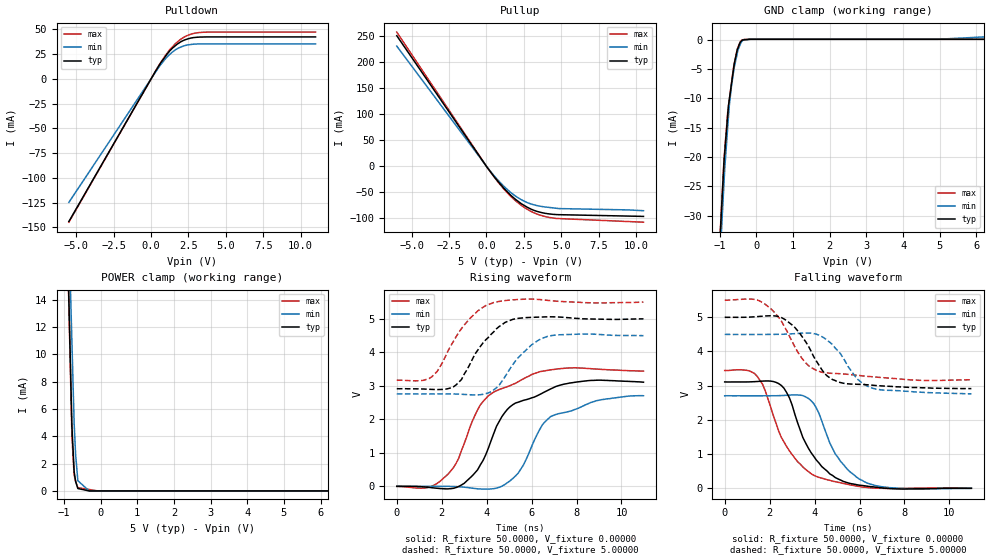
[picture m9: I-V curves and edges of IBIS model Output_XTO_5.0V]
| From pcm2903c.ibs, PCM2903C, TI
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[Model] Output_XTO_5.0V
Model_type Output
Vref  = 0.00000V
Cref  = 1.00000pF
Vmeas = 1.65000V
C_comp  2.00000pF 2.00000pF 2.00000pF
| variable   typ   min   max
[Voltage Range]   5.00000V  4.50000V  5.50000V
[POWER Clamp Reference]  5.00000V  4.50000V  5.50000V
[Pullup Reference]   5.00000V  4.50000V  5.50000V
[Pulldown Reference]   0.00000V  0.00000V  0.00000V
[GND Clamp Reference]   0.00000V  0.00000V  0.00000V
[Temperature Range]   25   85   -25
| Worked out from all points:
|   slope of the pulldown table from 0 to 0.75 V, typ, clamps not added: 40.8 ohm
|   slope of the pullup table from 0 to 0.75 V, typ, clamps not added: 26.9 ohm
|   GND clamp passes 1 mA (typ) near -0.48 V on its own axis
|   POWER clamp passes 1 mA (typ) near -0.70 V on its own axis
|   rising waveform, R_fixture 50.0000, V_fixture 0.00000: 20-80 % time 1.58ns typ, 1.62ns min, 1.54ns max; typ from 0 V to 3.11 V
|   falling waveform, R_fixture 50.0000, V_fixture 0.00000: 20-80 % time 1.37ns typ, 1.27ns min, 1.53ns max; typ from 3.11 V to 0 V
|   falling waveform, R_fixture 50.0000, V_fixture 5.00000: 20-80 % time 1.21ns typ, 1.2ns min, 1.3ns max; typ from 5 V to 2.92 V
|   rising waveform, R_fixture 50.0000, V_fixture 5.00000: 20-80 % time 1.28ns typ, 1.24ns min, 1.31ns max; typ from 2.92 V to 5 V
[GND Clamp]
-5V       -516.7mA   -511.3mA   -516.9mA
-881.1mV  -20.69mA   -24.2mA    -20.2mA
-861mV    -19.12mA   -21.83mA   -18.62mA
-780.2mV  -12.77mA   -14.83mA   -12.28mA
-760.1mV  -11.19mA   -13.08mA   -11.31mA
-739.6mV  -10.26mA   -11.31mA   -10.32mA
-679mV    -7.53mA    -7.887mA   -7.391mA
-623.5mV  -5.02mA    -5.556mA   -4.707mA
-522mV    -1.726mA   -2.33mA    -1.604mA
-380.7mV  -26.86uA   -130.3uA   -17.92uA
4.936V    100.6uA    99.12uA    98.92uA
10V       100.6uA    1.685mA    98.92uA
[Pulldown]
-5.5V     -144.1mA   -124.7mA   -144.7mA
279.4mV   7.251mA    6.327mA    7.216mA
658.9mV   16.41mA    14.59mA    16.72mA
1.063V    24.82mA    21.85mA    25.7mA
1.503V    31.88mA    27.93mA    33.47mA
1.902V    36.52mA    31.48mA    38.99mA
2.221V    39.05mA    33.32mA    42.17mA
2.6V      40.86mA    34.48mA    44.68mA
3.5V      42.18mA    35.22mA    46.98mA
11V       42.25mA    35.23mA    47.12mA
[Pullup]
-6V       250.4mA    230.5mA    257.3mA
39.2mV    -1.888mA   -1.438mA   -1.786mA
620.5mV   -23.75mA   -21.93mA   -24.46mA
1.121V    -40.74mA   -37.25mA   -42.2mA
1.621V    -55.47mA   -50.17mA   -57.51mA
2.081V    -66.41mA   -59.75mA   -69.29mA
2.698V    -78mA      -69.23mA   -81.85mA
3.139V    -83.99mA   -73.53mA   -88.61mA
3.557V    -87.78mA   -76.29mA   -93.35mA
4.301V    -91.58mA   -79.17mA   -98.42mA
4.837V    -92.68mA   -80.99mA   -100.1mA
10.5V     -95.98mA   -85.1mA    -107.1mA
[POWER Clamp]
-5V       474.9mA    423mA      493.3mA
-1.139V   44.73mA    45.92mA    45.58mA
-780.6mV  4.768mA    10.9mA     4.029mA
-719.7mV  1.418mA    4.948mA    1.152mA
-679.5mV  698.8uA    2.661mA    700.7uA
-618.7mV  176.3uA    747.4uA    239uA
-309.4mV  0A         0A         104.4uA
-38.05mV  0A         0A         0A
10V       0A         0A         0A
[Rising Waveform]
R_fixture = 50.0000
V_fixture = 0.00000
V_fixture_min = 0.00000
V_fixture_max = 0.00000
0s        0V         0V         0V
1.8ns     -57.41mV   546.8uV    89.3mV
2.52ns    -59.46mV   -4.152mV   557.5mV
3ns       89.55mV    -25.72mV   1.275V
3.72ns    642.5mV    -78.93mV   2.435V
4.44ns    1.795V     -52.7mV    2.856V
5.4ns     2.512V     389.9mV    3.123V
6.36ns    2.742V     1.698V     3.422V
6.84ns    2.907V     2.08V      3.478V
10.98ns   3.11V      2.705V     3.443V
[Falling Waveform]
R_fixture = 50.0000
V_fixture = 0.00000
V_fixture_min = 0.00000
V_fixture_max = 0.00000
0s        3.11V      2.705V     3.443V
1.44ns    3.122V     2.703V     3.279V
1.8ns     3.138V     2.706V     2.86V
2.52ns    3.007V     2.711V     1.489V
2.88ns    2.646V     2.724V     1.095V
3.96ns    937.5mV    2.48V      381.9mV
4.92ns    314.5mV    1.006V     192.3mV
6ns       89.87mV    266.5mV    50.41mV
7.32ns    -6.881mV   20.15mV    -4.144mV
10.98ns   0V         0V         0V
[Falling Waveform]
R_fixture = 50.0000
V_fixture = 5.00000
V_fixture_min = 4.50000
V_fixture_max = 5.50000
0s        5V         4.5V       5.5V
1.56ns    5.026V     4.498V     5.477V
2.16ns    5.043V     4.5V       5.182V
2.64ns    4.951V     4.505V     4.748V
3.48ns    4.402V     4.538V     3.765V
4.32ns    3.472V     4.437V     3.393V
5.04ns    3.11V      4.019V     3.353V
5.88ns    3.041V     3.21V      3.304V
6.36ns    3.025V     2.983V     3.273V
10.98ns   2.916V     2.76V      3.172V
[Rising Waveform]
R_fixture = 50.0000
V_fixture = 5.00000
V_fixture_min = 4.50000
V_fixture_max = 5.50000
0s        2.916V     2.76V      3.172V
1.56ns    2.896V     2.76V      3.272V
2.52ns    2.971V     2.759V     4.328V
2.88ns    3.189V     2.749V     4.712V
3.36ns    3.789V     2.732V     5.081V
4.32ns    4.618V     2.883V     5.49V
4.8ns     4.888V     3.257V     5.546V
5.64ns    5.031V     4.001V     5.588V
6.72ns    5.062V     4.481V     5.553V
10.98ns   5V         4.5V       5.5V
[Ramp]
| variable typ   min   max
dV/dt_r   1.86449/1.60590n  1.62277/1.59485n  2.06191/1.60414n
dV/dt_f   1.25365/1.23529n  1.04359/1.22682n  1.39757/1.27731n
R_load  =  50.0000Ohms
